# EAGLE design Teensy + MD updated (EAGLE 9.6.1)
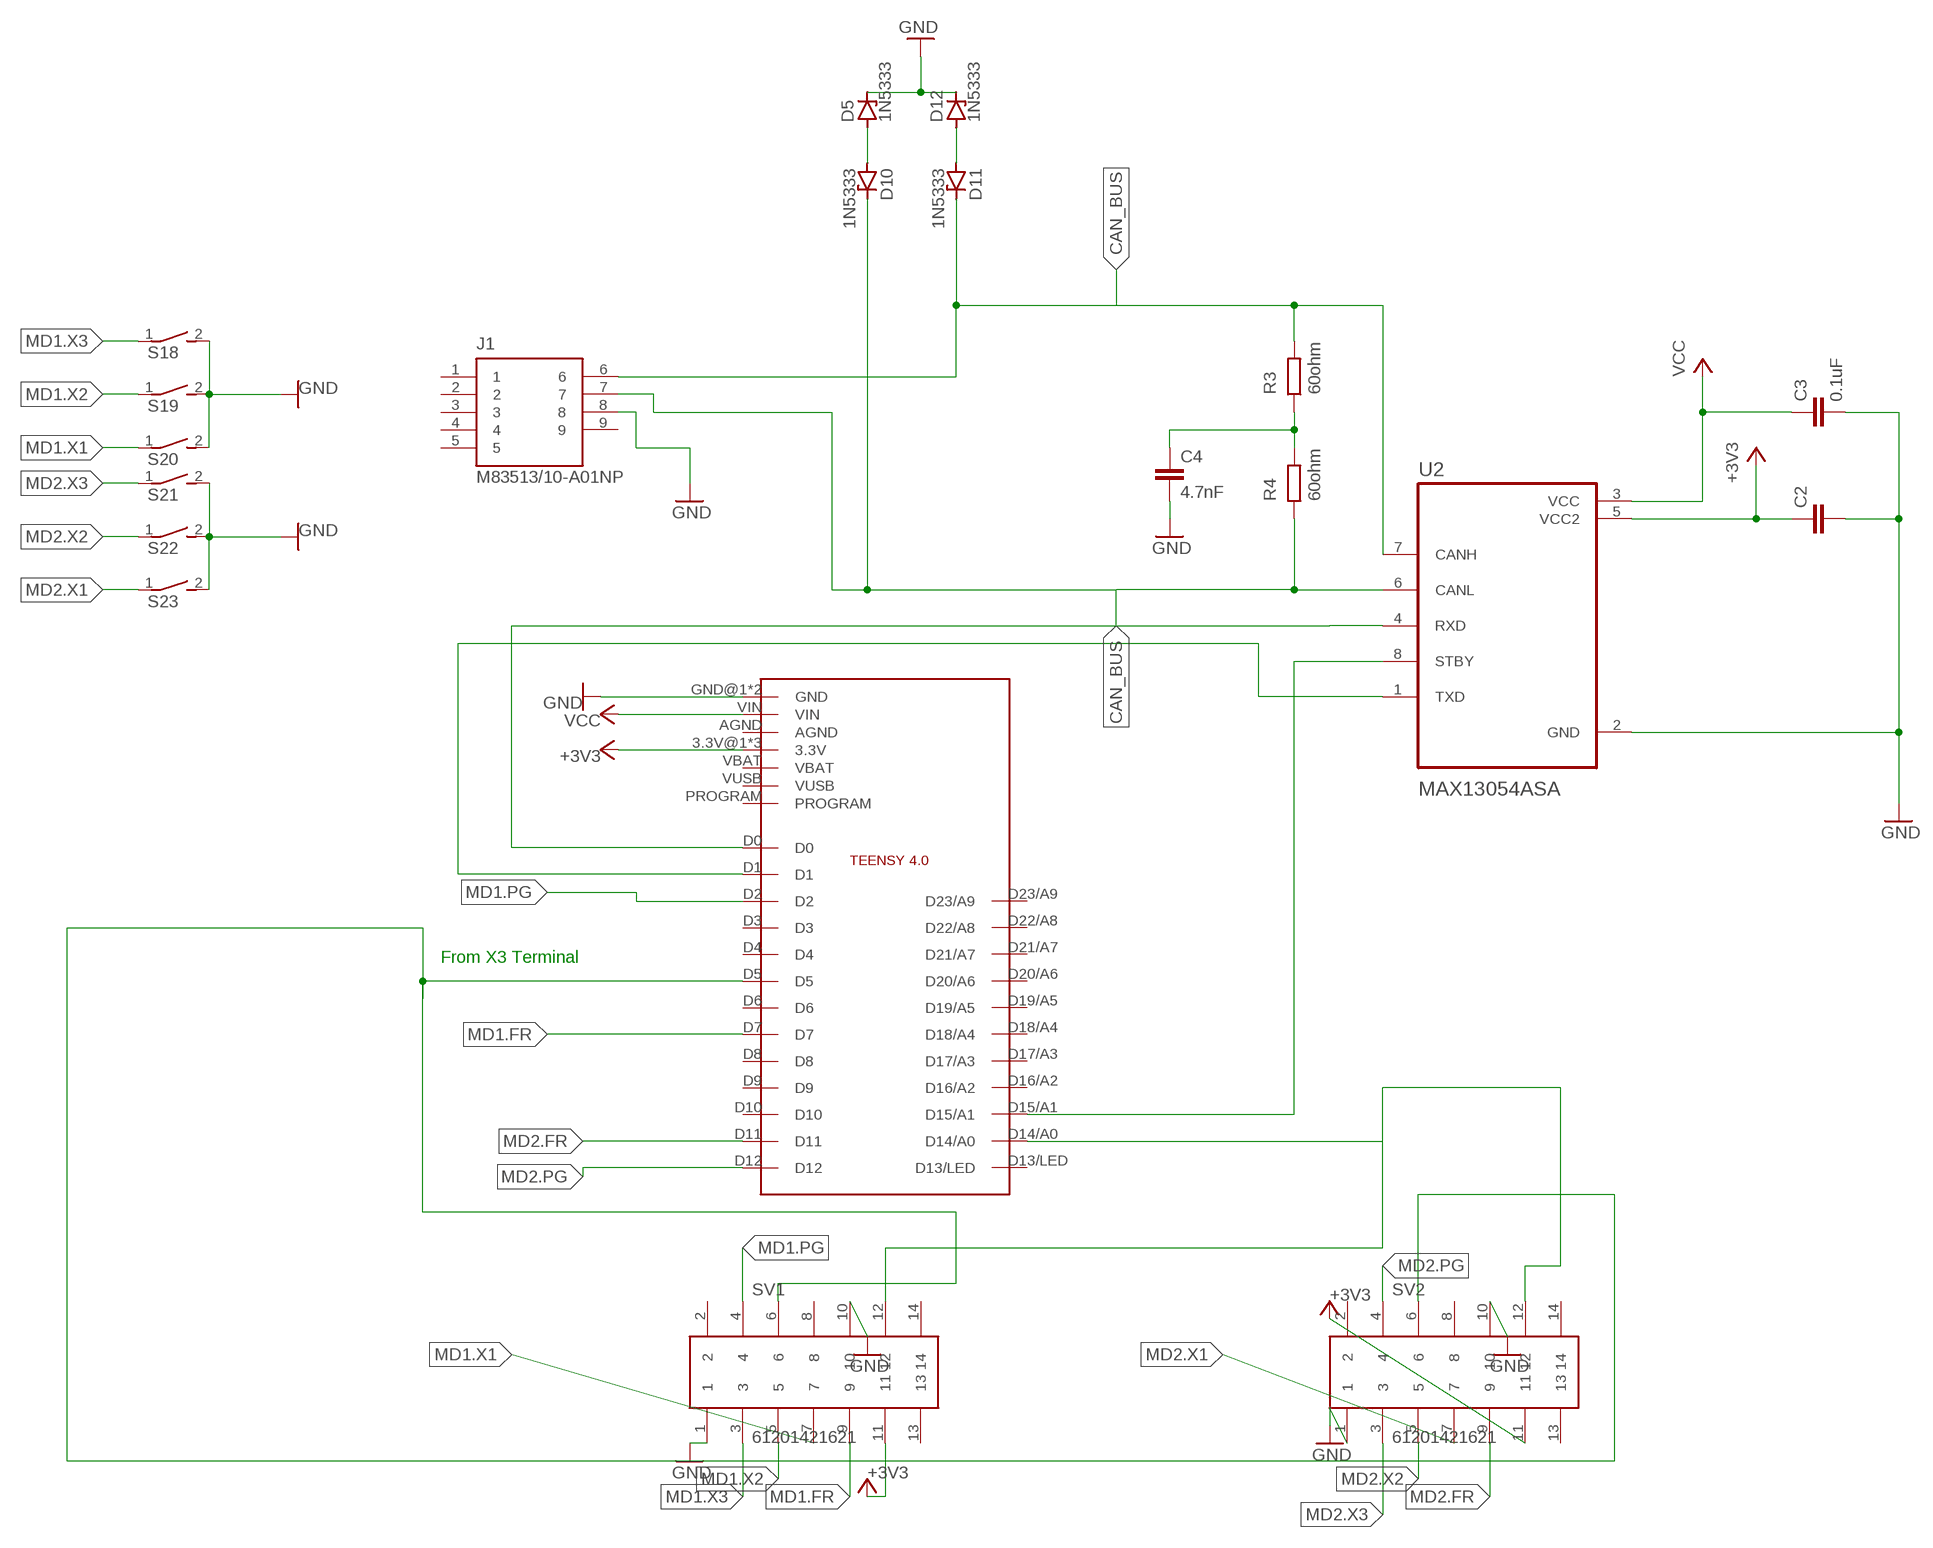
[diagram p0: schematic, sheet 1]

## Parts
C2  C2,5-3  [C2.5-3]
C3  0.1uF  C2,5-3  [C2.5-3]
C4  4.7nF  C2,5-3  [C2.5-3]
D5  1N5333  [C1702-15]
D10  1N5333  [C1702-15]
D11  1N5333  [C1702-15]
D12  1N5333  [C1702-15]
J1  M83513/10-A01NP  [BEL_M83513/10-A01NP]
R3  60ohm  R  (no package)
R4  60ohm  R  (no package)
S18  DS01E  [DS-01]
S19  DS01E  [DS-01]
S20  DS01E  [DS-01]
S21  DS01E  [DS-01]
S22  DS01E  [DS-01]
S23  DS01E  [DS-01]
SV1  61201421621  [61201421621]
SV2  61201421621  [61201421621]
U2  MAX13054ASA  [SOIC127P600X175-8N]
U$3  TEENSY4.0  [TEENSY4.0]

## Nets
+3V3: C2.1 SV1.11 SV2.11 U2.5(VCC2) U$3.3.3V@1(3.3V) U$3.3.3V@2(3.3V) U$3.ON/OFF(3.3V)
CAN_BUS: D11.C J1.6 R3.2 U2.7(CANH)
GND: C2.2 C3.2 C4.2 D5.C D12.C J1.8 S18.2 S19.2 S20.2 S21.2 S22.2 S23.2 SV1.1 SV1.10 SV2.1 SV2.10 U2.2(GND) U$3.GND@1(GND) U$3.GND@2(GND)
MD1.5V: SV1.6 SV2.6 U$3.D5
MD1.FR: SV1.9 U$3.D7
MD1.PG: SV1.4 U$3.D2
MD1.X1: S20.1 SV1.7
MD1.X2: S19.1 SV1.5
MD1.X3: S18.1 SV1.3
MD2.BK: SV1.12 SV2.12 U$3.D14/A0
MD2.FR: SV2.9 U$3.D11
MD2.PG: SV2.4 U$3.D12
MD2.X1: S23.1 SV2.7
MD2.X2: S22.1 SV2.5
MD2.X3: S21.1 SV2.3
N$9: D10.C J1.7 R4.1 U2.6(CANL)
N$10: U2.8(STBY) U$3.D15/A1
N$11: U2.4(RXD) U$3.D0
N$12: U2.1(TXD) U$3.D1
N$13: C4.1 R3.1 R4.2
N$14: D5.A D10.A
N$15: D11.A D12.A
VCC: C3.1 U2.3(VCC) U$3.VIN
Unconnected: J1.1 J1.2 J1.3 J1.4 J1.5 J1.9 SV1.2 SV1.8 SV1.13 SV1.14 SV2.2 SV2.8 SV2.13 SV2.14 U$3.AGND U$3.D3 U$3.D4 U$3.D6 U$3.D8 U$3.D9 U$3.D10 U$3.D13/LED U$3.D16/A2 U$3.D17/A3 U$3.D18/A4 U$3.D19/A5 U$3.D20/A6 U$3.D21/A7 U$3.D22/A8 U$3.D23/A9 U$3.PROGRAM U$3.VBAT U$3.VUSB

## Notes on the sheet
- From X3 Terminal

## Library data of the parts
C2-C4 = capacitor-wima:C: CAPACITOR
D5 D10-D12 = diode:1N5333: Z DIODE
J1 = M83513_10-A01NP:M83513/10-A01NP: MIL-DTL-83513 PCB Mounted Connector | Plug | 9 Positions | Shell Finish - Cadmium | Male | PCB Solder Pins | 0.109in (2.77 mm) Pin Length; AVAILABILITY: Unavailable; DESCRIPTION: MIL-DTL-83513 PCB Mounted Connector | Plug | 9 Positions | Shell Finish - Nickel | Male | PCB Solder Pins | 0.109 (2.77 mm) Pin Length | Jackpost Attached; MF: Cinch Connectivity Solutions; MP: M83513/10-A01NP; PACKAGE: None; PRICE: None
R3 R4 = ngspice-simulation:R: RESISTOR
S18-S23 = switch-dil:DS01E: DIL/CODE SWITCH; OC_FARNELL: unknown; OC_NEWARK: unknown
SV1 SV2 = Wuerth_Elektronik_eiCan_05_Box_Header_IDC_Connectors_1_2:61201421621: WR-BHD 2.54mm Male Box Header, 14 Pins
U2 = MAX13054ASA:MAX13054ASA; DESCRIPTION: 1/1 Transceiver Full CANbus 8-SOIC; DIGI-KEY_PART_NUMBER: MAX13054ASA+TTR-ND; DIGI-KEY_PURCHASE_URL: https://www.digikey.com/product-detail/en/maxim-integrated/MAX13054ASA-T/MAX13054ASA-TTR-ND/1475460?utm_source=snapeda&utm_medium=aggregator&utm_campaign=symbol; MF: Maxim Integrated; MP: MAX13054ASA+; PACKAGE: SOIC-8 Maxim
U$3 = Teensy4.0:TEENSY4.0

## Module RESISTER
Ports: 

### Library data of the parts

## Module GND
Ports: 

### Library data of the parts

## Module MOTOR
Ports: 

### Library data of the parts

## Module MOTORDRIVER
Ports: U(io) V(io) W(io) VCC(io) GND(io) 5V(io) GND1(io) HA(io) HB(io) HC(io) RS232(io) PWR(io) ALM(io) GND2(io) ALM1(io) X3(io) PG(io) X2(io) 5V1(io) X1(io) 5V2(io) PR(io) GND3(io) EN(io) BR(io)

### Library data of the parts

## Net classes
0 default: width 0.305 mm, drill 0.508 mm, clearance 0.254 mm

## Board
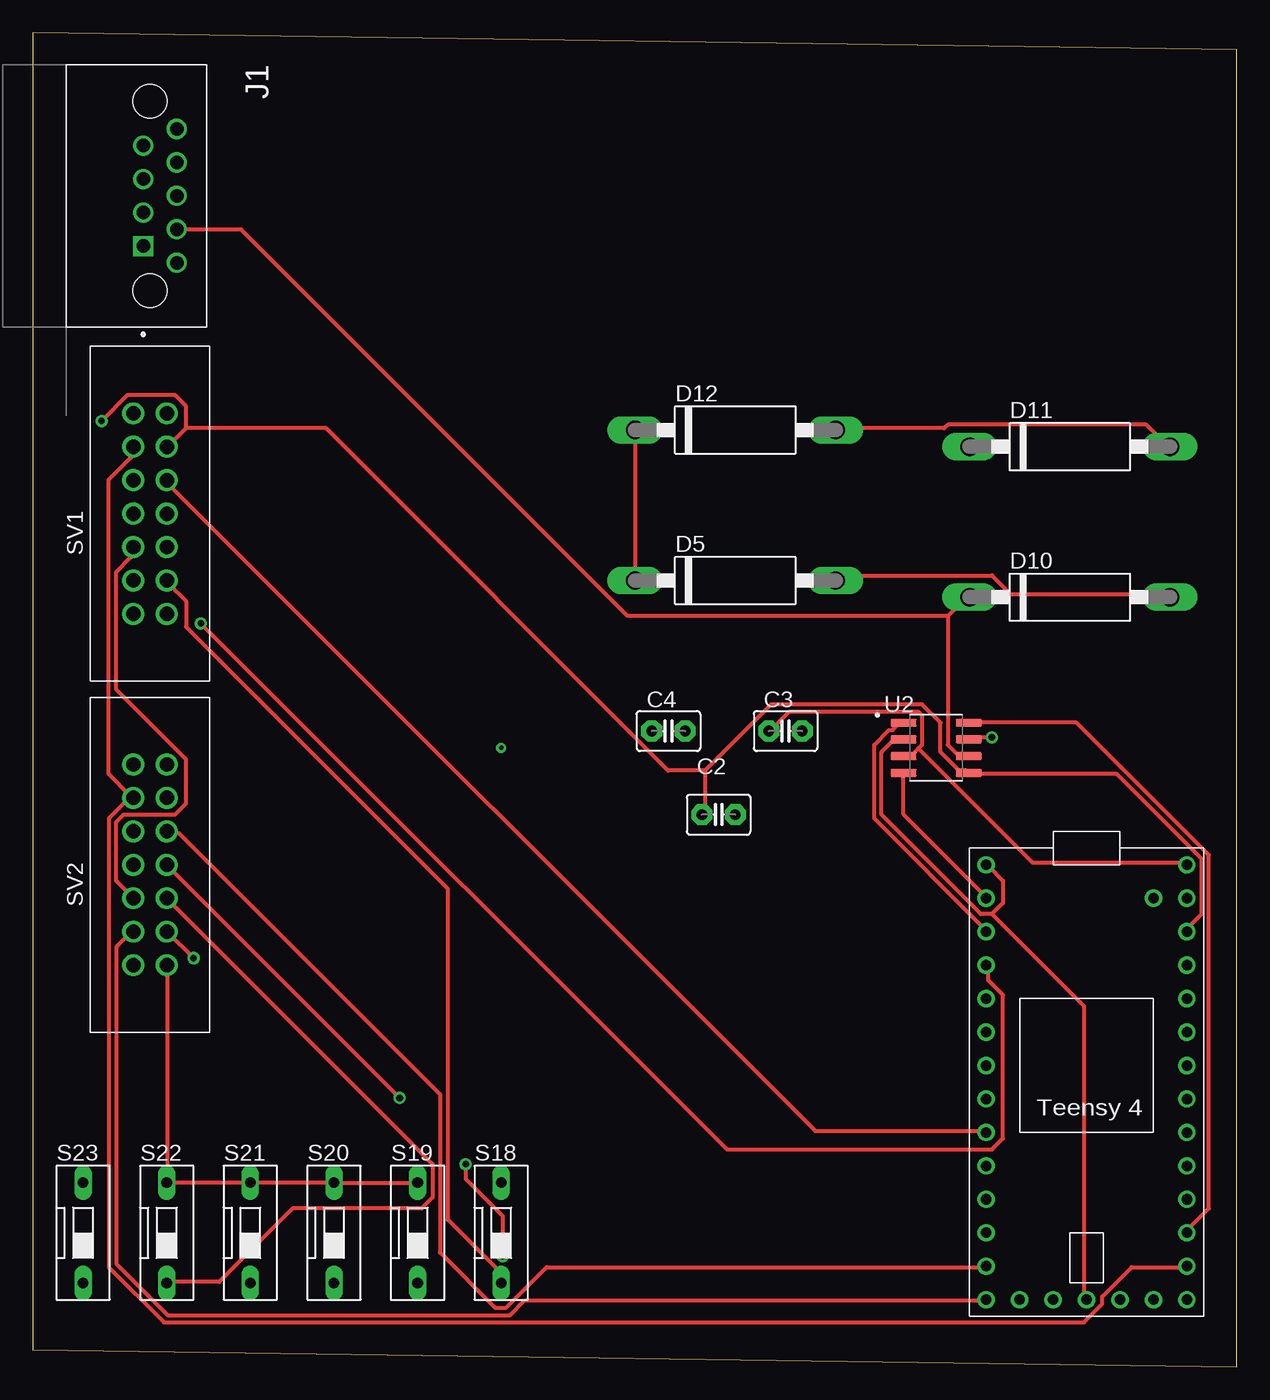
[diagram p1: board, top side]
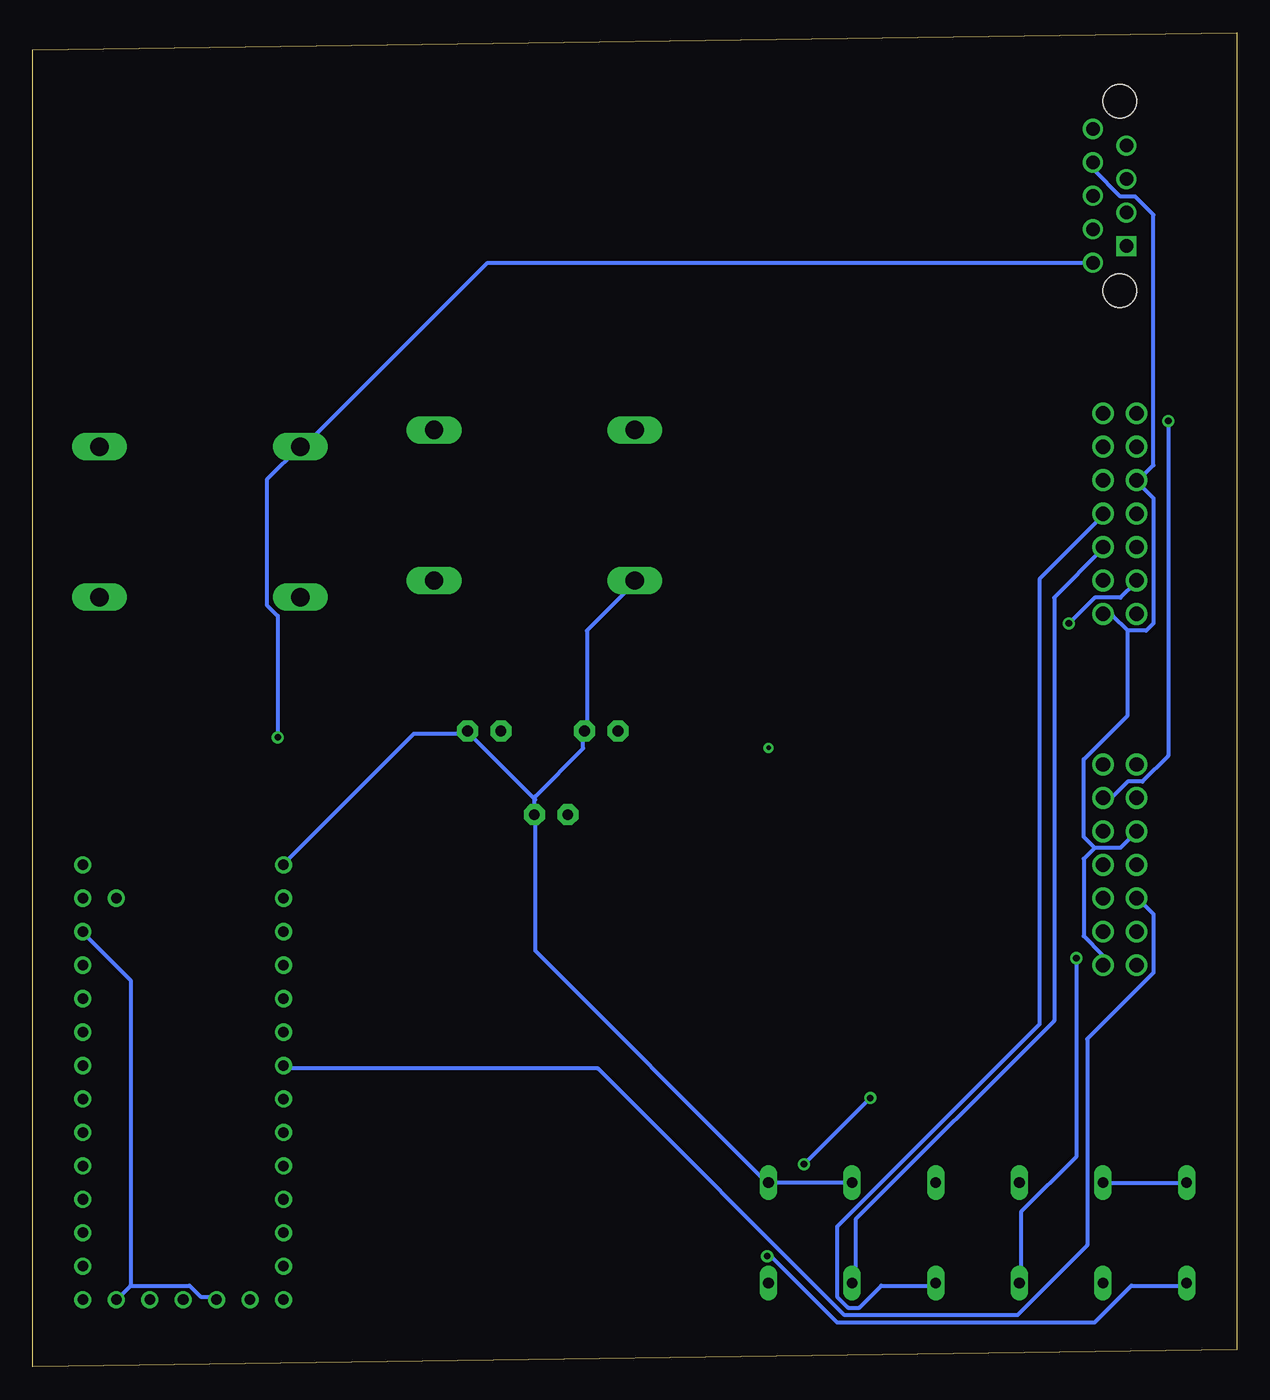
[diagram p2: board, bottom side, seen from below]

Size 91.42 x 101.27 mm. Coordinates in mm from the lower left corner, seen from the top.
Outline: 0,1.27 91.42,0 91.42,100 0,101.27 0,1.27
Copper layers (1*16): Top 0.035mm / dielectric 1.5mm / Bottom 0.035mm
Design rules "default": minimum track width 6mil, minimum drill 0.35mm, track to track 6mil, track to pad 6mil, pad to pad 6mil, via to via 6mil, smd to smd 6mil, copper to edge 40mil, drill to drill 6mil, minimum pad ring 10mil, minimum via ring 8mil, stop-mask expansion 4mil, vias tented up to drill 0mil, thermal gap 10mil

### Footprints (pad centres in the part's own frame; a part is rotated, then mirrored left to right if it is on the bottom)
C2.5-3 = drill 0.813 pad 1.6 octagon: 1 -1.27,0; 2 1.27,0
C1702-15 = drill 1.397 long: A 7.62,0; C -7.62,0
BEL_M83513/10-A01NP = drill 1.02 square: 1 3.81,-0.508 | drill 1.02: 2 1.27,-0.508; 3 0,2.032; 4 -1.27,-0.508; 5 -3.81,-0.508; 6 5.08,2.032; 7 2.54,2.032; 8 -2.54,2.032; 9 -5.08,2.032 | hole 2.57: -7.188,0; 7.188,0
DS-01 = drill 0.813 long: 1 0,-3.81; 2 0,3.81
61201421621 = drill 1.1: 1 -2.54,-1.27; 2 -2.54,1.27; 3 0,-1.27; 4 0,1.27; 5 2.54,-1.27; 6 2.54,1.27; 7 5.08,-1.27; 8 5.08,1.27; 9 7.62,-1.27; 10 7.62,1.27; 11 10.16,-1.27; 12 10.16,1.27; 13 12.7,-1.27; 14 12.7,1.27
SOIC127P600X175-8N = smd 1.97 x 0.59: 1 -2.475,1.905; 2 -2.475,0.635; 3 -2.475,-0.635; 4 -2.475,-1.905; 5 2.475,-1.905; 6 2.475,-0.635; 7 2.475,0.635; 8 2.475,1.905
TEENSY4.0 = drill 0.8: 3.3V@1 7.62,10.16; 3.3V@2 -2.54,-17.78; AGND 7.62,12.7; D0 -7.62,12.7; D1 -7.62,10.16; D2 -7.62,7.62; D3 -7.62,5.08; D4 -7.62,2.54; D5 -7.62,0; D6 -7.62,-2.54; D7 -7.62,-5.08; D8 -7.62,-7.62; D9 -7.62,-10.16; D10 -7.62,-12.7; D11 -7.62,-15.24; D12 -7.62,-17.78; D13/LED 7.62,-17.78; D14/A0 7.62,-15.24; D15/A1 7.62,-12.7; D16/A2 7.62,-10.16; D17/A3 7.62,-7.62; D18/A4 7.62,-5.08; D19/A5 7.62,-2.54; D20/A6 7.62,0; D21/A7 7.62,2.54; D22/A8 7.62,5.08; D23/A9 7.62,7.62; GND@1 -7.62,15.24; GND@2 0,-17.78; ON/OFF 5.08,-17.78; PROGRAM 2.54,-17.78; VBAT -5.08,-17.78; VIN 7.62,15.24; VUSB 5.08,12.7

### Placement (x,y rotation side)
C2  52.07,41.91 0 top
C3  57.15,48.26 0 top
C4  48.26,48.26 0 top
D5  53.34,59.69 0 top
D10  78.74,58.42 0 top
D11  78.74,69.85 0 top
D12  53.34,71.12 0 top
J1  8.89,88.9 270 top
S18  35.56,10.16 0 top
S19  29.21,10.16 0 top
S20  22.86,10.16 0 top
S21  16.51,10.16 0 top
S22  10.16,10.16 0 top
S23  3.81,10.16 0 top
SV1  8.89,59.69 90 top
SV2  8.89,33.02 90 top
U2  68.58,46.99 0 top
U$3  80.01,22.86 0 top

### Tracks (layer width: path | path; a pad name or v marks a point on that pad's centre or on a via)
+3V3  (via drill 0.51)
  Top 0.305: v5.21,71.81 7.16,73.76 10.79,73.76 11.63,72.92 11.63,71.25 | 11.63,71.25 10.24,69.85 SV1.11 | U$3.3.3V@1 87.63,33.25 88.75,34.37 88.75,38.56 82.32,44.98 71.14,44.98 U2.5 70.87,45.26 70.31,45.26 68.91,46.66 68.91,48.9 67.51,50.29 56.06,50.29 51.03,45.26 | 51.03,45.26 51.03,41.91 C2.1 | 11.63,71.25 22.25,71.25 48.23,45.26 51.03,45.26
  Bottom 0.305: v5.21,71.81 5.21,46.38 7.16,44.42 8.28,44.42 9.4,43.31 9.96,43.31 SV2.11 | 84,6.15 79.53,6.15 78.69,5.31 77.57,5.31 U$3.3.3V@2 | 84,6.15 84.84,5.31 U$3.ON/OFF | 84,6.15 84,29.34 87.63,32.97 U$3.3.3V@1
CAN_BUS  (via drill 0.51)
  Top 0.305: 70.51,47.62 U2.7 71.14,47.78 v72.82,47.78
  Bottom 0.305: v72.82,47.78 72.82,57 73.66,57.84 73.66,67.33 71.14,69.85 D11.C 70.87,69.85 56.9,83.82 J1.6
GND
  Top 0.305: 66.65,47.62 U2.2 65.84,47.5 65.28,47.5 64.44,46.66 64.44,41.91 71.98,34.37 72.82,34.37 | D12.C D5.C | 72.82,34.37 73.66,35.2 73.66,36.88 72.54,38 U$3.GND@1 | 72.82,34.37 79.81,27.38 79.81,5.31 U$3.GND@2 | S19.2 S20.2 S21.2 10.24,13.97 | 10.24,13.97 10.24,30.45 SV2.1 | 10.24,13.97 S22.2
  Bottom 0.305: 53.34,43.03 C2.2 53.26,41.91 53.26,31.57 35.66,13.97 S18.2 S19.2 | 53.34,43.03 53.34,43.18 53.26,43.31 49.63,46.94 49.63,48.06 C4.2 49.35,48.34 49.35,55.88 45.72,59.51 D5.C | 53.34,43.03 53.26,43.03 58.29,48.06 C3.2 58.57,48.06 62.48,48.06 72.26,38.28 U$3.GND@1 | J1.8 10.79,91.36 10.79,90.81 8.84,88.85 7.72,88.85 6.32,87.45 6.32,68.45 7.44,67.33 SV1.10 7.44,67.06 6.32,65.94 6.32,56.44 6.88,55.88 8.28,55.88 | 8.28,55.88 9.4,57 9.96,57 SV1.1 | 10.79,39.4 11.63,38.56 11.63,32.69 10.24,31.29 10.24,30.73 SV2.1 | 10.79,39.4 8.84,39.4 7.72,40.51 SV2.10 | S22.2 S23.2 | 8.28,55.88 8.28,49.45 11.63,46.1 11.63,40.23 10.79,39.4
MD1.5V
  Top 0.305: SV1.6 7.44,62.03 7.44,61.47 6.32,60.35 6.32,51.41 11.63,46.1 11.63,42.75 10.79,41.91 6.88,41.91 6.32,41.35 6.32,36.88 7.44,35.76 SV2.6
  Bottom 0.305: U$3.D5 72.26,22.63 48.51,22.63 29.79,3.91 16.66,3.91 11.35,9.22 11.35,24.87 6.32,29.9 6.32,34.37 7.44,35.48 SV2.6
MD1.FR
  Top 0.305: U$3.D7 72.26,17.88 59.41,17.88 10.24,67.06 SV1.9
MD1.PG  (via drill 0.51)
  Top 0.305: v12.75,56.44 52.7,16.48 72.82,16.48 73.66,17.32 73.66,28.22 72.54,29.34 72.54,30.45 U$3.D2
  Bottom 0.305: v12.75,56.44 10.79,58.4 8.84,58.4 7.72,59.51 SV1.4
MD1.X1
  Bottom 0.305: S20.1 23.09,6.15 27,6.15 28.68,4.47 29.52,4.47 30.35,5.31 30.35,10.62 14.99,25.98 14.99,59.79 10.24,64.54 SV1.7
MD1.X2
  Bottom 0.305: S19.1 28.96,6.43 28.96,11.18 13.87,26.26 13.87,58.4 10.24,62.03 SV1.5
MD1.X3
  Top 0.305: S18.1 35.38,6.43 35.38,7.26 31.47,11.18 31.47,36.32 11.63,56.16 11.63,58.12 10.24,59.51 SV1.3
MD2.BK
  Top 0.305: 7.44,43.31 5.77,41.63 5.77,7.54 9.96,3.35 79.81,3.35 81.2,4.75 81.2,5.31 83.44,7.54 87.63,7.54 U$3.D14/A0 | 7.44,43.31 5.77,44.98 5.77,67.33 7.44,69.01 7.44,69.85 SV1.12 | 7.44,43.31 SV2.12
MD2.FR
  Top 0.305: U$3.D11 72.26,7.54 39.01,7.54 35.94,4.47 35.1,4.47 30.91,8.66 30.91,20.68 11.07,40.51 10.24,40.51 SV2.9
MD2.PG
  Top 0.305: U$3.D12 72.26,5.03 37.34,5.03 36.22,3.91 10.24,3.91 6.32,7.82 6.32,31.85 7.44,32.97 SV2.4
MD2.X1  (via drill 0.51)
  Top 0.305: v35.66,8.38 35.66,11.46 32.87,14.25 v32.87,15.37 | v27.84,20.4 10.24,38 SV2.7
  Bottom 0.305: v35.66,8.38 35.38,8.38 30.35,3.35 10.79,3.35 8,6.15 3.81,6.15 S23.1 | v27.84,20.4 v32.87,15.37
MD2.X2
  Top 0.305: SV2.5 30.35,15.37 30.35,12.85 29.52,12.01 19.74,12.01 14.15,6.43 10.24,6.43 S22.1
MD2.X3  (via drill 0.51)
  Top 0.305: v12.19,31.01 10.24,32.97 SV2.3
  Bottom 0.305: v12.19,31.01 12.19,15.93 16.38,11.73 16.38,6.43 S21.1
N$1  (via drill 0.35)
  other vias: 35.56,46.99
N$9
  Top 0.305: 71.6,46.35 U2.6 70.87,46.38 70.31,46.38 69.47,47.22 69.47,57 | 69.47,57 70.87,58.4 D10.C | 69.47,57 45.16,57 15.82,86.33 11.07,86.33 J1.7
  Bottom 0.305: D10.C 70.07,58.42
N$10
  Top 0.305: U2.8 79.25,48.9 89.31,38.84 89.31,12.01 87.63,10.34 U$3.D15/A1
N$11
  Top 0.305: U2.4 66.12,44.98 66.12,41.91 72.26,35.76 U$3.D0
N$12
  Top 0.305: U2.1 65.84,48.9 65.28,48.34 65,48.34 63.88,47.22 63.88,41.63 72.26,33.25 U$3.D1
N$14
  Top 0.305: D10.A 86.23,58.67 74.22,58.67 72.82,60.07 61.37,60.07 61.09,59.79 D5.A
  Bottom 0.305: D5.A 62.01,59.69
N$15
  Top 0.305: D12.A 61.09,71.25 69.19,71.25 69.47,71.53 84.56,71.53 86.23,69.85 D11.A
  Bottom 0.305: D11.A 85.31,69.85 | 62.19,71.3 62.03,71.14 | 62.03,71.14 62.01,71.12 | 62.03,71.14 61.92,71.25 61.09,71.25 D12.A
VCC
  Top 0.305: 65.56,46.35 U2.3 66.12,46.38 66.67,46.38 67.23,46.94 | 67.23,46.94 67.51,47.22 67.51,49.45 67.23,49.73 57.45,49.73 56.06,48.34 C3.1 | 67.23,46.94 75.89,38.28 87.63,38.28 U$3.VIN

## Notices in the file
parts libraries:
Wuerth_Elektronik_eiCan_05_Box_Header_ID: Copyright: Würth Elektronik
